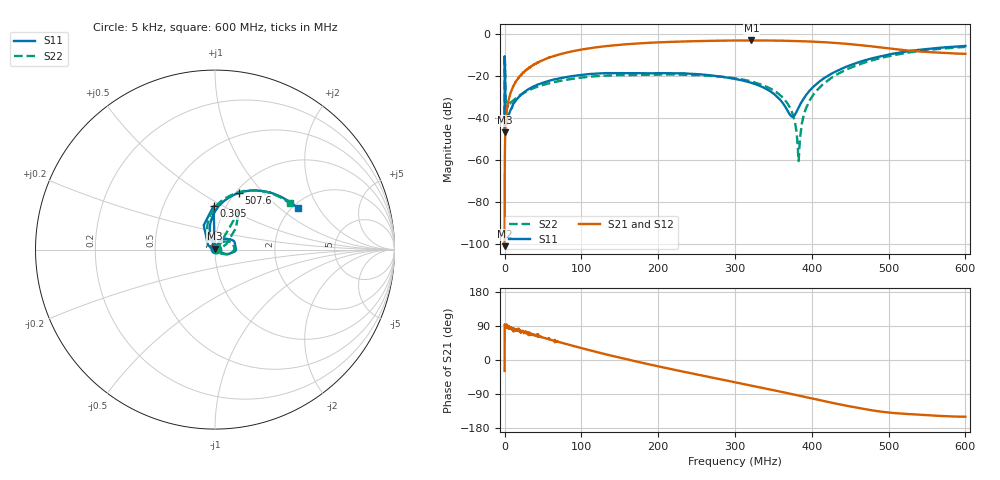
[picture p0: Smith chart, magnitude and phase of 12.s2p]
#  HZ  S  MA  R  50.00
! Rohde & Schwarz Vector Network Analyzer
! Rohde-Schwarz,ZNL6-2Port,1323001206101378,1.50.1.34-21.10.1.104
! Created: UTC 1/22/2024, 9:02:53 AM
! freq[Hz]  mag:S11  ang:S11  mag:S21  ang:S21  mag:S12  ang:S12  mag:S22  ang:S22
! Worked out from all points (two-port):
!   6000 points, 5 kHz to 600 MHz, reference 50 ohm
!   highest |S21| = -3.13 dB at 321.5 MHz (marker M1); lowest = -100.9 dB at 5 kHz (marker M2)
!   |S21| within 3 dB of the highest: 124.8 MHz to 482.4 MHz (357.6 MHz wide, 118 % of centre)
!   lowest |S11| = -46.8 dB at 5 kHz (marker M3), VSWR 1.01, Z = 49.9 + j0.434 ohm
!   |S11| at or under -10 dB: start of sweep to 497.6 MHz
!   |S22| runs from -60.5 to -6.2 dB; largest |S21 - S12| = 0.044
!   S11 on the Smith chart (normalised r, x): 5 kHz: 1.00, +0.01; 305 kHz: 0.88, +0.45; 507.6 MHz: 1.04, +0.74; 600 MHz: 2.14, +1.34
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5000  0.004563 107.6  8.979e-06 -28.9  4.332e-05 -50.7  0.01202 12.0
305047.5  0.2424 91.9  0.001358 92.9  0.00138 86.8  0.2532 58.2
3105491  0.007748 61.9  0.016 87.6  0.01595 86.5  0.01851 17.6
4405697  0.01008 64.3  0.02261 86.3  0.02239 86.0  0.0197 21.9
8806394  0.0169 64.5  0.04403 85.6  0.045 81.0  0.02424 31.5
1.64076e7  0.02851 66.2  0.08224 79.3  0.08165 78.1  0.03124 39.7
4.531217e7  0.06436 56.7  0.2176 61.9  0.2163 61.0  0.05738 44.3
1.000208e8  0.106 31.6  0.4236 31.4  0.4211 30.0  0.09123 28.5
2.000367e8  0.1162 3.7  0.6279 -16.8  0.626 -17.7  0.1077 7.2
3.000525e8  0.08478 -15.3  0.695 -58.8  0.6924 -59.6  0.0881 -14.8
3.214559e8  0.06835 -21.0  0.6971 -67.8  0.6946 -68.7  0.07371 -21.0
3.484602e8  0.04017 -22.9  0.6934 -78.9  0.6902 -80.2  0.04744 -29.5
3.66263e8  0.01746 -6.5  0.6851 -86.6  0.682 -87.9  0.02507 -37.2
3.755645e8  0.01075 47.8  0.6788 -90.7  0.6758 -92.1  0.01158 -43.7
3.826656e8  0.01753 91.3  0.673 -93.8  0.6702 -95.3  0.001001 -117.5
3.846659e8  0.02068 96.9  0.6713 -94.7  0.6683 -96.1  0.003268 153.3
3.902668e8  0.03066 105.5  0.6659 -97.2  0.663 -98.6  0.013 137.8
4.000683e8  0.05082 109.9  0.6552 -101.5  0.652 -102.9  0.03171 130.5
4.371742e8  0.1439 100.8  0.5964 -117.4  0.594 -118.6  0.1202 111.3
5.000842e8  0.3231 70.8  0.45 -138.6  0.4457 -139.7  0.2936 78.3
5.075854e8  0.3433 67.0  0.4332 -140.1  0.43 -141.0  0.3135 74.2
6e8  0.5156 26.6  0.3362 -149.8  0.3371 -150.4  0.4904 31.6
